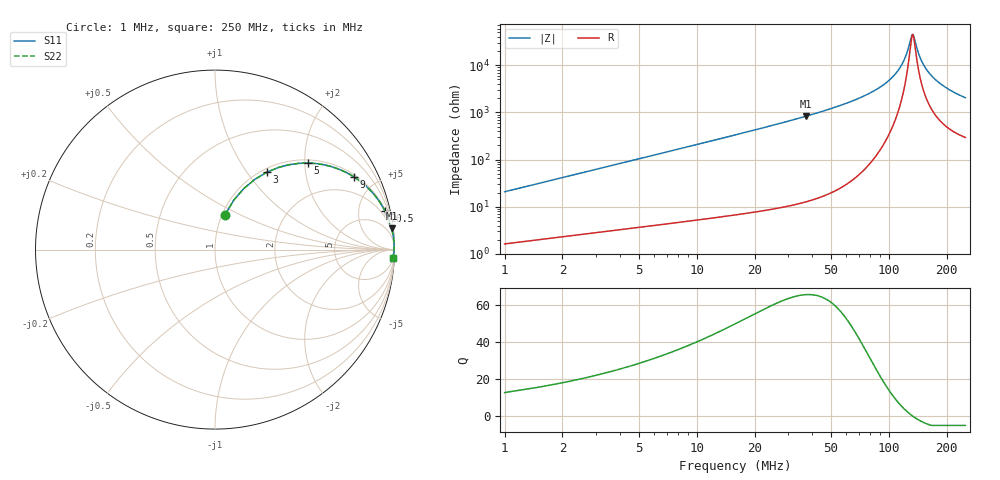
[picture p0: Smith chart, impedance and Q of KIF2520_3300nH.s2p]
!version-2
!date-12.2020
!Series
# MHz S RI R 50
!Freq ReS11 ImS11 ReS21 ImS21 ReS12 ImS12 ReS22 ImS22
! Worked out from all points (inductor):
!   499 points, 1 MHz to 250 MHz, reference 50 ohm
!   read as one part in series: L = 3.3 uH near 2 MHz
!   highest Q = 65.4 at 37 MHz (marker M1), where L = 3.58 uH
!   self-resonance near 133 MHz
!   S11 on the Smith chart (normalised r, x): 1 MHz: 1.03, +0.41; 3 MHz: 1.06, +1.24; 5 MHz: 1.07, +2.08; 9 MHz: 1.10, +3.75; 20.5 MHz: 1.16, +8.71; 250 MHz: 7, -41
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1  0.0554 0.1927  0.9446 -0.1927  0.9446 -0.1927  0.0554 0.1927
3  0.2882 0.4308  0.7118 -0.4308  0.7118 -0.4308  0.2882 0.4308
5  0.5184 0.4824  0.4816 -0.4824  0.4816 -0.4824  0.5184 0.4824
7  0.6747 0.4538  0.3253 -0.4538  0.3253 -0.4538  0.6747 0.4538
9  0.7727 0.4062  0.2273 -0.4062  0.2273 -0.4062  0.7727 0.4062
13.5  0.8837 0.3099  0.1163 -0.3099  0.1163 -0.3099  0.8837 0.3099
20.5  0.9464 0.2164  0.0536 -0.2164  0.0536 -0.2164  0.9464 0.2164
37  0.984 0.1181  0.016 -0.1181  0.016 -0.1181  0.984 0.1181
42.5  0.9882 0.1005  0.0118 -0.1005  0.0118 -0.1005  0.9882 0.1005
84  0.9975 0.0344  0.00246 -0.0344  0.00246 -0.0344  0.9975 0.0344
110.5  0.9981 0.0135  0.00187 -0.0135  0.00187 -0.0135  0.9981 0.0135
119  0.9981 0.00805  0.00194 -0.00805  0.00194 -0.00805  0.9981 0.00805
125.5  0.998 0.0042  0.00204 -0.0042  0.00204 -0.0042  0.998 0.0042
131  0.9978 0.00111  0.00217 -0.00111  0.00217 -0.00111  0.9978 0.00111
133.5  0.9978 -0.000253  0.00223 0.000253  0.00223 0.000253  0.9978 -0.000253
142  0.9975 -0.00469  0.00249 0.00469  0.00249 0.00469  0.9975 -0.00469
147.5  0.9973 -0.00743  0.00269 0.00743  0.00269 0.00743  0.9973 -0.00743
156  0.997 -0.0115  0.00303 0.0115  0.00303 0.0115  0.997 -0.0115
167  0.9965 -0.0164  0.00355 0.0164  0.00355 0.0164  0.9965 -0.0164
185  0.9955 -0.024  0.00453 0.024  0.00453 0.024  0.9955 -0.024
208.5  0.994 -0.0331  0.00604 0.0331  0.00604 0.0331  0.994 -0.0331
250  0.9907 -0.0475  0.00926 0.0475  0.00926 0.0475  0.9907 -0.0475
